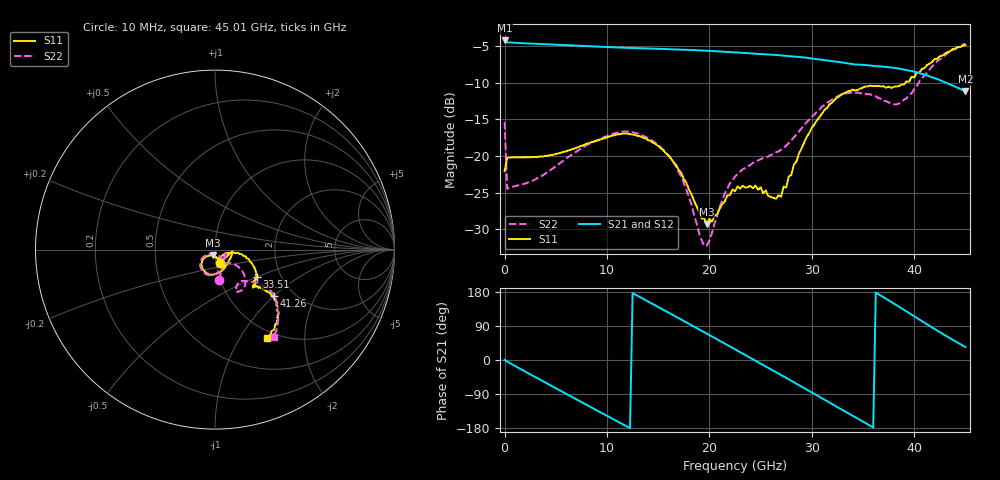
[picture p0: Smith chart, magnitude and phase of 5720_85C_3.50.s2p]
! Device:  ADRF5720
! Description: 0.5dB LSB GaAs MMIC 6-bit Digital Attenuator
! Frequency:  0.000009 -  40 GHz
! Ports:
!	RF1	= Port 1
!	RF2	= Port 2
! Vdd:  3.3 Volt
! Vss:  -3.3 Volt
! Control:  0/3.3 Volt
! State:  3.50 dB attenuation
! Data:  The device was measured using G-S-G Probes on a matrix board.
!  Data was collected using an calibrated 4 port network analyzer.
!  The reference plane for this measurement is at the launchers.
! Note:  Analog Devices supplies this data as a sample of measured data
!  for this product.  Your particular data for this product may vary.
!  Data was taken at 85 degrees C.
!  Analog Devices reserves the right to change this data at anytime.
# GHZ S DB R 45.0
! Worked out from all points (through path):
!   181 points, 10 MHz to 45.01 GHz, reference 45 ohm
!   highest |S21| = -4.24 dB at 10 MHz (marker M1); lowest = -11.2 dB at 45.01 GHz (marker M2)
!   group delay of S21, straight-line fit = 42.1 ps
!   lowest |S11| = -29.3 dB at 19.76 GHz (marker M3), VSWR 1.07, Z = 43.9 - j2.85 ohm
!   |S11| at or under -10 dB: start of sweep to 39.15 GHz
!   |S22| runs from -32.3 to -4.7 dB; largest |S21 - S12| = 0.003
!   S11 on the Smith chart (normalised r, x): 10 MHz: 1.05, -0.16; 33.51 GHz: 1.51, -0.49; 41.26 GHz: 1.58, -1.00; 45.01 GHz: 0.91, -1.32
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0.01  -22.06 -69.1  -4.24 0.3  -4.22 0.3  -15.38 -81.8
0.26  -20.28 -6.0  -4.50 -4.0  -4.49 -4.0  -24.49 -7.5
2.26  -20.19 -22.8  -4.65 -34.1  -4.63 -34.0  -23.65 -23.5
4.26  -19.97 -42.4  -4.77 -63.5  -4.75 -63.5  -22.16 -45.4
7.76  -18.51 -66.6  -4.99 -114.6  -4.97 -114.6  -18.75 -72.0
11.51  -16.97 -98.1  -5.23 -169.0  -5.21 -168.9  -16.69 -103.5
13.26  -17.33 -114.3  -5.31 165.6  -5.29 165.7  -17.07 -119.0
15.26  -18.97 -131.4  -5.39 136.3  -5.37 136.4  -18.84 -136.1
17.26  -22.32 -142.3  -5.49 106.8  -5.47 107.0  -22.85 -148.2
19.26  -28.55 -121.2  -5.61 77.1  -5.59 77.3  -31.53 -117.9
19.76  -29.30 -108.8  -5.65 69.6  -5.63 69.8  -32.23 -90.7
21.51  -26.21 -74.8  -5.78 43.5  -5.77 43.7  -25.11 -52.6
22.76  -24.15 -72.4  -5.89 24.8  -5.87 25.0  -22.49 -52.8
24.76  -24.65 -71.4  -6.07 -5.3  -6.05 -5.0  -20.62 -54.6
27.01  -25.58 -32.0  -6.28 -39.5  -6.26 -39.2  -19.15 -43.0
30.26  -15.71 -12.9  -6.75 -89.7  -6.73 -89.5  -14.37 -38.1
33.51  -11.17 -33.0  -7.36 -139.7  -7.34 -139.4  -11.42 -54.1
35.76  -10.41 -43.3  -7.67 -174.3  -7.65 -174.0  -11.61 -63.1
37.76  -10.72 -43.1  -7.94 153.4  -7.92 153.8  -12.76 -56.2
39.26  -9.81 -41.5  -8.29 128.1  -8.27 128.4  -12.15 -45.5
41.26  -7.59 -38.5  -9.02 94.2  -9.00 94.5  -8.63 -36.5
45.01  -4.86 -59.4  -11.16 34.4  -11.13 34.7  -4.66 -56.1
